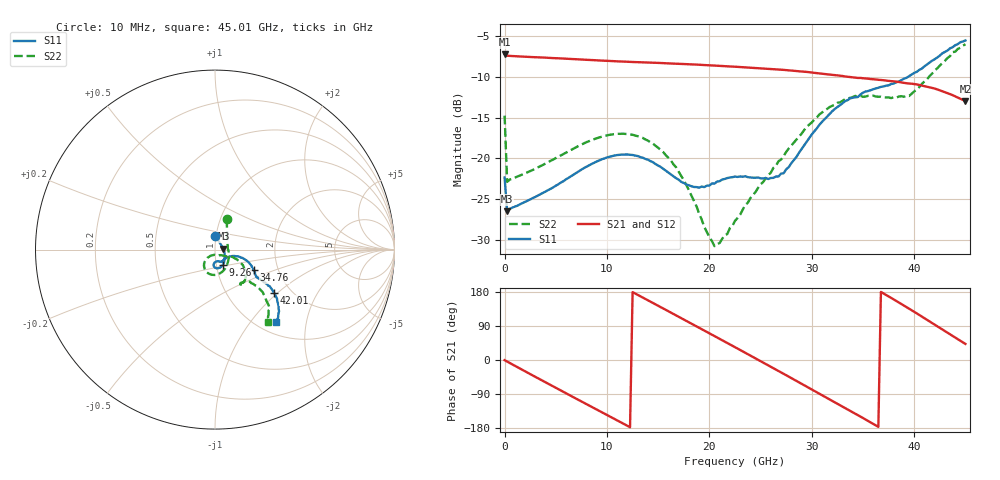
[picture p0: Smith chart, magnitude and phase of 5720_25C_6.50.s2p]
! Device:  ADRF5720
! Description: 0.5dB LSB GaAs MMIC 6-bit Digital Attenuator
! Frequency:  0.000009 -  40 GHz
! Ports:
!	RF1	= Port 1
!	RF2	= Port 2
! Vdd:  3.3 Volt
! Vss:  -3.3 Volt
! Control:  0/3.3 Volt
! State:  6.50 dB attenuation
! Data:  The device was measured using G-S-G Probes on a matrix board.
!  Data was collected using an calibrated 4 port network analyzer.
!  The reference plane for this measurement is at the launchers.
! Note:  Analog Devices supplies this data as a sample of measured data
!  for this product.  Your particular data for this product may vary.
!  Data was taken at 25 degrees C.
!  Analog Devices reserves the right to change this data at anytime.
# GHZ S DB R 45.0
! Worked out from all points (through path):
!   181 points, 10 MHz to 45.01 GHz, reference 45 ohm
!   highest |S21| = -7.20 dB at 10 MHz (marker M1); lowest = -13.0 dB at 45.01 GHz (marker M2)
!   group delay of S21, straight-line fit = 41.3 ps
!   lowest |S11| = -26.5 dB at 260 MHz (marker M3), VSWR 1.10, Z = 49.4 + j0.587 ohm
!   |S11| at or under -10 dB: start of sweep to 39.39 GHz
!   |S22| runs from -30.8 to -6.0 dB; largest |S21 - S12| = 0.00048
!   S11 on the Smith chart (normalised r, x): 10 MHz: 0.99, +0.15; 9.26 GHz: 1.07, -0.19; 34.76 GHz: 1.50, -0.37; 42.01 GHz: 1.64, -0.94; 45.01 GHz: 1.21, -1.36
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0.01  -22.37 88.5  -7.20 -0.5  -7.20 -0.5  -14.76 69.3
0.26  -26.53 7.2  -7.39 -4.1  -7.39 -4.1  -22.91 3.5
2.01  -25.37 -13.8  -7.51 -29.9  -7.51 -29.9  -21.86 -16.7
4.26  -23.92 -32.3  -7.64 -62.5  -7.64 -62.5  -20.48 -37.8
6.01  -22.59 -43.5  -7.75 -87.8  -7.75 -87.8  -19.30 -52.0
7.76  -21.21 -54.4  -7.87 -113.0  -7.87 -113.0  -18.16 -65.6
9.26  -20.27 -64.1  -7.97 -134.4  -7.97 -134.4  -17.44 -77.2
12.26  -19.58 -83.4  -8.15 -177.3  -8.15 -177.3  -17.07 -100.8
15.26  -21.08 -95.0  -8.29 139.5  -8.29 139.5  -18.98 -122.9
18.01  -23.33 -87.1  -8.44 99.6  -8.44 99.6  -23.93 -132.8
20.51  -23.12 -70.2  -8.60 63.1  -8.60 63.1  -30.82 -94.3
22.76  -22.30 -63.4  -8.76 30.2  -8.76 30.2  -27.36 -46.0
24.76  -22.37 -55.1  -8.92 0.7  -8.92 0.8  -23.65 -32.5
26.76  -22.25 -36.9  -9.09 -29.0  -9.09 -29.0  -20.37 -24.2
28.51  -19.84 -20.7  -9.27 -55.2  -9.28 -55.2  -17.70 -24.3
30.26  -16.69 -16.4  -9.49 -81.6  -9.49 -81.6  -15.24 -28.7
32.26  -13.94 -20.8  -9.77 -111.6  -9.78 -111.6  -13.39 -37.5
34.76  -12.15 -27.9  -10.12 -149.3  -10.13 -149.2  -12.32 -49.9
37.76  -10.87 -33.7  -10.51 163.9  -10.51 164.0  -12.60 -52.4
39.51  -9.90 -33.4  -10.81 135.6  -10.82 135.6  -12.35 -47.8
42.01  -7.82 -36.2  -11.43 93.1  -11.43 93.1  -9.20 -41.6
45.01  -5.51 -49.8  -12.96 42.4  -12.96 42.4  -5.98 -53.6
